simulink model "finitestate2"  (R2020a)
settings: Solver=FixedStepDiscrete  StartTime=0.0  StopTime=100  RelTol=1e-3  EnableMultiTasking=on

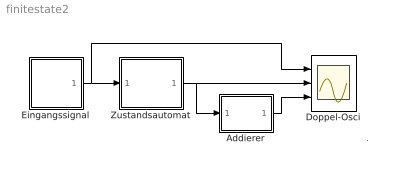
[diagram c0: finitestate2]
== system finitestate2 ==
  note: .
  Addierer : Subsystem
  Doppel-Osci : Scope  NumInputPorts=3
  Eingangssignal : Subsystem  mask(Zufallsereignis){p=0.3}
      mask prompts: p "Wahrscheinlichkeit"
      mask help: Erzeugt Zufallsfolge aus 0/1 mit vorgegebener Wahrscheinlichkeit fuer 1
  Zustandsautomat : Subsystem
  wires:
  Eingangssignal/1(Out) -> Doppel-Osci/1, Zustandsautomat/1(In)
  Zustandsautomat/1(Out) -> Doppel-Osci/2, Addierer/1(In)
  Addierer/1(Out) -> Doppel-Osci/3

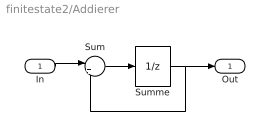
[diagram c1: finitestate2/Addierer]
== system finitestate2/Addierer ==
  In : Inport
  Sum : Sum  Inputs=|++
  Summe : UnitDelay  SampleTime=-1  HasFrameUpgradeWarning=on
  Out : Outport
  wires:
  Summe/1 -> Sum/2, Out/1
  Sum/1 -> Summe/1
  In/1 -> Sum/1

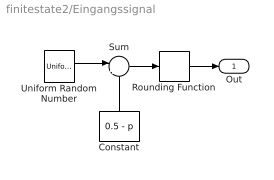
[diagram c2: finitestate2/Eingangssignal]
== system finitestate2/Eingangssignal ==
  Constant : Constant  Value=0.5 - p
  Rounding Function : Rounding  Operator=round
  Sum : Sum  Inputs=|+-
  Uniform Random Number : UniformRandomNumber  Minimum=0  SampleTime=1
  Out : Outport
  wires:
  Rounding Function/1 -> Out/1
  Uniform Random Number/1 -> Sum/1
  Sum/1 -> Rounding Function/1
  Constant/1 -> Sum/2

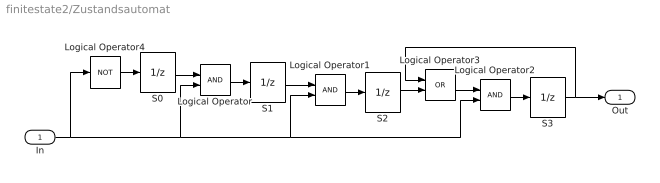
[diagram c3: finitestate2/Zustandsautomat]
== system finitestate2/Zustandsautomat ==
  In : Inport
  Logical Operator : Logic
  Logical Operator1 : Logic
  Logical Operator2 : Logic
  Logical Operator3 : Logic  Operator=OR
  Logical Operator4 : Logic  Operator=NOT
  S0 : UnitDelay  InitialCondition=1  SampleTime=-1  HasFrameUpgradeWarning=on
  S1 : UnitDelay  SampleTime=-1  HasFrameUpgradeWarning=on
  S2 : UnitDelay  SampleTime=-1  HasFrameUpgradeWarning=on
  S3 : UnitDelay  SampleTime=-1  HasFrameUpgradeWarning=on
  Out : Outport
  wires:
  S0/1 -> Logical Operator/1
  Logical Operator/1 -> S1/1
  S1/1 -> Logical Operator1/1
  Logical Operator1/1 -> S2/1
  Logical Operator2/1 -> S3/1
  S3/1 -> Logical Operator3/1, Out/1
  S2/1 -> Logical Operator3/2
  Logical Operator3/1 -> Logical Operator2/1
  Logical Operator4/1 -> S0/1
  In/1 -> Logical Operator4/1, Logical Operator2/2, Logical Operator1/2, Logical Operator/2
